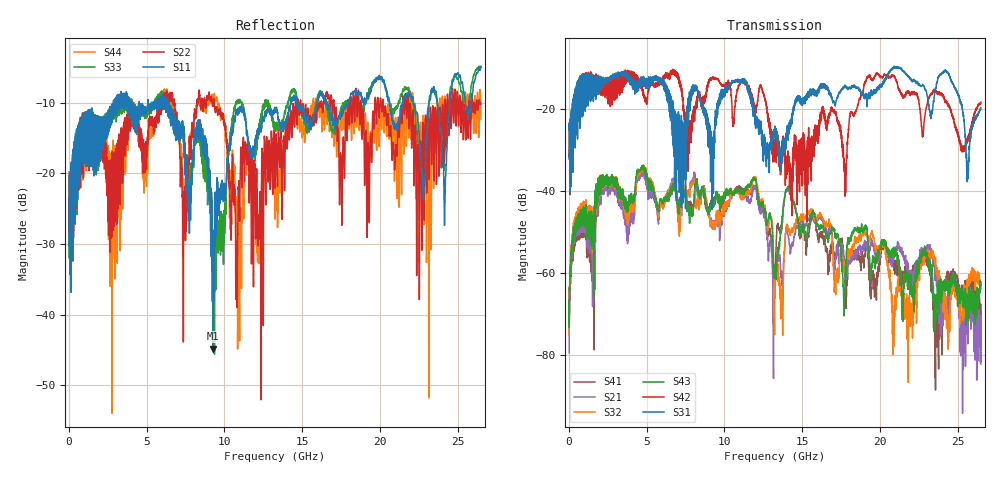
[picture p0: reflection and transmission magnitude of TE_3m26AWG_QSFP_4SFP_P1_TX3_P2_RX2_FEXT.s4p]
!Agilent Technologies,N5222A,MY51421691,A.10.00.00
!Agilent N5222A: A.10.00.00
!Date: Friday, January 30, 2015 12:37:43
!Correction: S11(Full 4 Port(1,2,3,4))
!S12(Full 4 Port(1,2,3,4))
!S13(Full 4 Port(1,2,3,4))
!S14(Full 4 Port(1,2,3,4))
!S21(Full 4 Port(1,2,3,4))
!S22(Full 4 Port(1,2,3,4))
!S23(Full 4 Port(1,2,3,4))
!S24(Full 4 Port(1,2,3,4))
!S31(Full 4 Port(1,2,3,4))
!S32(Full 4 Port(1,2,3,4))
!S33(Full 4 Port(1,2,3,4))
!S34(Full 4 Port(1,2,3,4))
!S41(Full 4 Port(1,2,3,4))
!S42(Full 4 Port(1,2,3,4))
!S43(Full 4 Port(1,2,3,4))
!S44(Full 4 Port(1,2,3,4))
!S4P File: Measurements: <S11,S12,S13,S14>,
!<S21,S22,S23,S24>,
!<S31,S32,S33,S34>,
!<S41,S42,S43,S44>:
# Hz S  dB  R 50.0
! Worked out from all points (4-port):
!   2650 points, 10 MHz to 26.5 GHz, reference 50 ohm
!   strongest paths, dB at 10 MHz, 6.63 GHz, 13.26 GHz, 19.88 GHz, 26.5 GHz:
!     S31: -25.0, -17.7, -24.7, -15.2, -19.6
!     S42: -24.7, -11.3, -30.3, -11.5, -18.2
!     S43: -66.7, -39.4, -59.4, -54.3, -63.0
!     S32: -75.2, -38.6, -66.1, -54.3, -62.2
!     S21: -79.5, -38.3, -59.5, -56.3, -82.3
!     S41: -68.5, -39.4, -61.4, -60.8, -71.3
!   lowest |S11| = -44.8 dB at 9.27 GHz (marker M1), VSWR 1.01, Z = 49.8 + j0.552 ohm
!   |S11| at or under -10 dB: start of sweep to 2.858 GHz; 6.4 GHz to 14.26 GHz (7.855 GHz wide, 76.1 % of centre); 16.59 GHz to 17.98 GHz (1.384 GHz wide, 8.01 % of centre)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
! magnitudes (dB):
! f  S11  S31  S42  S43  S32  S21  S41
! 10 MHz  -20.7  -25.0  -24.7  -66.7  -75.2  -79.5  -68.5
! 2.3 GHz  -12.2  -12.6  -12.4  -38.0  -38.0  -39.3  -39.2
! 9.27 GHz  -44.8  -27.7  -12.1  -43.3  -48.3  -47.9  -42.0
! 10.97 GHz  -11.2  -12.8  -14.0  -40.2  -40.7  -39.8  -38.8
! 13.65 GHz  -13.0  -35.3  -32.7  -48.4  -67.0  -61.2  -49.5
! 15.58 GHz  -13.1  -16.7  -33.0  -45.7  -44.6  -45.6  -46.8
! 26.5 GHz  -4.8  -19.6  -18.2  -63.0  -62.2  -82.3  -71.3
